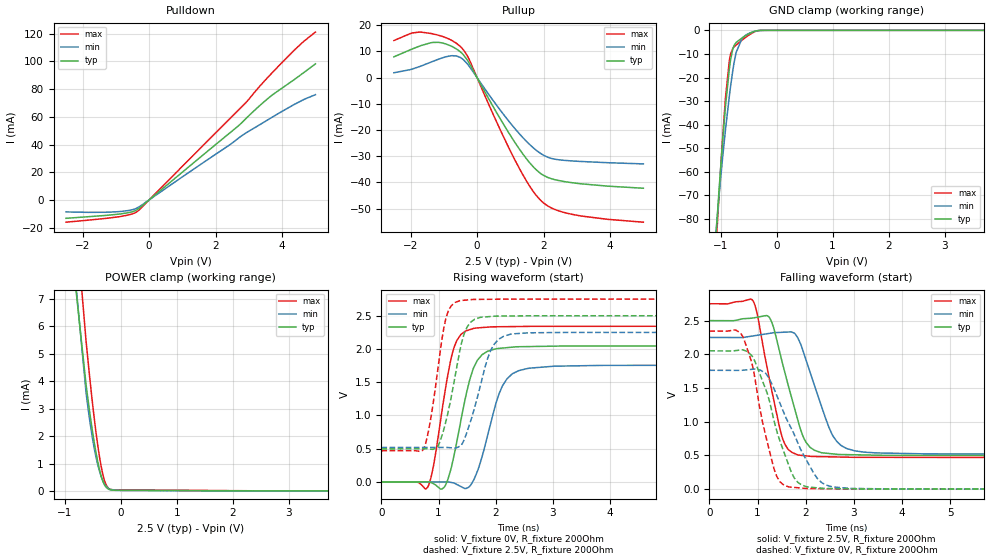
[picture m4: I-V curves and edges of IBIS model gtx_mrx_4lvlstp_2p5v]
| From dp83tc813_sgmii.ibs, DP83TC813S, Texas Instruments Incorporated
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| gtx_mrx_4lvlstp_2p5v
[Model]   gtx_mrx_4lvlstp_2p5v
Model_type   I/O
Polarity   Non-Inverting
Enable   Active-Low
Vinl = 0.7
Vinh = 1.7
Vmeas = 1.25
Vref = 1.25
Cref = 2pF
Rref = 100000
|   typ   min   max
C_comp   2.97pF   2.92pF   3pF
[Voltage Range]   2.5   2.25   2.75
[Temperature Range]   27   150   -40
[Pullup Reference]   2.5   2.25   2.75
[Pulldown Reference]   0   0   0
[Power Clamp Reference]   2.5   2.25   2.75
[GND Clamp Reference]   0   0   0
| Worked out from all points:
|   slope of the pulldown table from 0 to 0.375 V, typ, clamps not added: 49.7 ohm
|   slope of the pullup table from 0 to 0.375 V, typ, clamps not added: 43.5 ohm
|   GND clamp passes 1 mA (typ) near -0.45 V on its own axis
|   POWER clamp passes 1 mA (typ) near -0.40 V on its own axis
|   falling waveform, V_fixture 2.5V, R_fixture 200Ohm: 20-80 % time 449ps typ, 502ps min, 384ps max; typ from 2.5 V to 0.498 V
|   rising waveform, V_fixture 0V, R_fixture 200Ohm: 20-80 % time 310ps typ, 349ps min, 269ps max; typ from 0 V to 2.05 V
|   rising waveform, V_fixture 2.5V, R_fixture 200Ohm: 20-80 % time 281ps typ, 338ps min, 230ps max; typ from 0.498 V to 2.5 V
|   falling waveform, V_fixture 0V, R_fixture 200Ohm: 20-80 % time 537ps typ, 689ps min, 404ps max; typ from 2.05 V to 0 V
[Pulldown]
|   Voltage   I(typ)   I(min)   I(max)
-2.5V     -13.29mA   -8.687mA   -16.1mA
-925mV    -10.31mA   -8.492mA   -12.22mA
-512.5mV  -8.603mA   -7.139mA   -10.18mA
-347.5mV  -6.835mA   -5.631mA   -8.211mA
2.638V    52.57mA    43.69mA    63.75mA
2.885V    58.13mA    47.96mA    69.7mA
3.462V    71.02mA    56.29mA    85.76mA
3.958V    80.11mA    63.42mA    98.27mA
4.633V    91.66mA    72.28mA    114.2mA
5V        98.27mA    76.01mA    121.2mA
[GND Clamp]
|   Voltage   I(typ)   I(min)   I(max)
-2.5V     -648.4mA   -555.8mA   -723.6mA
-1.097V   -92.72mA   -89.85mA   -98.54mA
-1.03V    -68.88mA   -71.01mA   -71.09mA
-962.5mV  -46.81mA   -53.8mA    -45.43mA
-917.5mV  -33.73mA   -43.36mA   -30.37mA
-835mV    -14.9mA    -26.33mA   -11.67mA
-782.5mV  -8.005mA   -17.22mA   -7.74mA
-722.5mV  -5.155mA   -9.439mA   -6.239mA
-617.5mV  -3.266mA   -3.489mA   -4.19mA
-497.5mV  -1.539mA   -1.362mA   -2.076mA
-265mV    -17.6uA    -39uA      -18.83uA
5V        0A         0A         0A
[Pullup]
|   Voltage   I(typ)   I(min)   I(max)
-2.5V     7.944mA    1.866mA    14.16mA
-1.938V   11mA       3.316mA    17.07mA
-1.323V   13.44mA    6.242mA    16.69mA
-752.5mV  11.89mA    8.383mA    14.16mA
-460mV    9.358mA    7.341mA    11.34mA
-257.5mV  5.988mA    4.704mA    7.488mA
642.5mV   -14.55mA   -11.48mA   -18.41mA
1.272V    -27.27mA   -21.43mA   -34.67mA
1.677V    -33.87mA   -26.64mA   -43.23mA
2.007V    -37.38mA   -29.68mA   -47.93mA
2.953V    -40.27mA   -31.88mA   -52.42mA
5V        -42.22mA   -32.93mA   -55.18mA
[POWER Clamp]
|   Voltage   I(typ)   I(min)   I(max)
-2.5V     111.6mA    76.29mA    155.1mA
-1.06V    12.33mA    13.14mA    16.14mA
-617.5mV  3.849mA    3.558mA    5.431mA
-557.5mV  2.922mA    2.624mA    4.207mA
-505mV    2.182mA    1.927mA    3.214mA
-445mV    1.436mA    1.271mA    2.191mA
-392.5mV  892.8uA    818.2uA    1.42mA
-347.5mV  528.8uA    520.2uA    876.1uA
-302.5mV  272.9uA    303.6uA    464.8uA
-257.5mV  124.4uA    163.1uA    204.9uA
-212.5mV  57.82uA    83.72uA    84.66uA
5V        0A         0A         0A
[Ramp]
R_load = 200
|   typ   min   max
dV/dt_r   1.22962/3.0687e-10   1.05646/3.46896e-10   1.40614/2.68578e-10
dV/dt_f   1.20079/4.50432e-10   1.03862/4.9969e-10   1.36802/3.84068e-10
[Falling Waveform]
V_fixture = 2.5V
V_fixture_min = 2.25V
V_fixture_max = 2.75V
R_fixture = 200Ohm
C_fixture = 0F
|   Time   V(typ)   V(min)   V(max)
0s        2.499V     2.249V     2.749V
911.3ps   2.538V     2.272V     2.786V
996.1ps   2.549V     2.282V     2.591V
1.296ns   2.476V     2.315V     1.464V
1.536ns   1.817V     2.327V     721.1mV
1.838ns   1.023V     2.243V     508.3mV
2.084ns   626.4mV    1.75V      488.1mV
2.54ns    524.8mV    825.3mV    479.1mV
3.013ns   510mV      569.2mV    472.2mV
12ns      497.8mV    518.2mV    468.9mV
[Rising Waveform]
V_fixture = 0V
V_fixture_min = 0V
V_fixture_max = 0V
R_fixture = 200Ohm
C_fixture = 0F
|   Time   V(typ)   V(min)   V(max)
0s        104.9uV    168.7uV    95.35uV
808.8ps   191.3uV    308.5uV    -79.75mV
917.9ps   -29.34mV   327.3uV    271.4mV
1.093ns   -84.93mV   357.6uV    1.251V
1.205ns   158.4mV    -4.326mV   1.799V
1.319ns   601.2mV    -36.71mV   2.125V
1.612ns   1.71V      22.82mV    2.307V
2.115ns   2.012V     1.437V     2.333V
2.557ns   2.035V     1.705V     2.338V
12ns      2.049V     1.761V     2.344V
[Rising Waveform]
V_fixture = 2.5V
V_fixture_min = 2.25V
V_fixture_max = 2.75V
R_fixture = 200Ohm
C_fixture = 0F
|   Time   V(typ)   V(min)   V(max)
0s        497.8mV    518.2mV    468.9mV
738.4ps   498.6mV    518.7mV    492.6mV
833.5ps   496.3mV    518.8mV    807mV
981.6ps   524.4mV    518.9mV    1.653V
1.121ns   885mV      519mV      2.43V
1.377ns   1.988V     539.9mV    2.726V
1.558ns   2.398V     907.1mV    2.739V
1.916ns   2.487V     1.981V     2.746V
2.268ns   2.495V     2.222V     2.748V
12ns      2.499V     2.249V     2.749V
[Falling Waveform]
|Gnd
V_fixture = 0V
V_fixture_min = 0V
V_fixture_max = 0V
R_fixture = 200Ohm
C_fixture = 0F
|   Time   V(typ)   V(min)   V(max)
0s        2.051V     1.762V     2.344V
693.8ps   2.066V     1.763V     2.262V
963.8ps   1.864V     1.78V      1.568V
1.102ns   1.608V     1.747V     1.004V
1.347ns   1.003V     1.483V     293.6mV
1.63ns    392.4mV    1.002V     37.61mV
1.833ns   105.2mV    694.4mV    21.62mV
2.173ns   24.19mV    231.1mV    8.727mV
2.577ns   9.329mV    31.95mV    4.466mV
12ns      104.7uV    169.7uV    95.18uV
